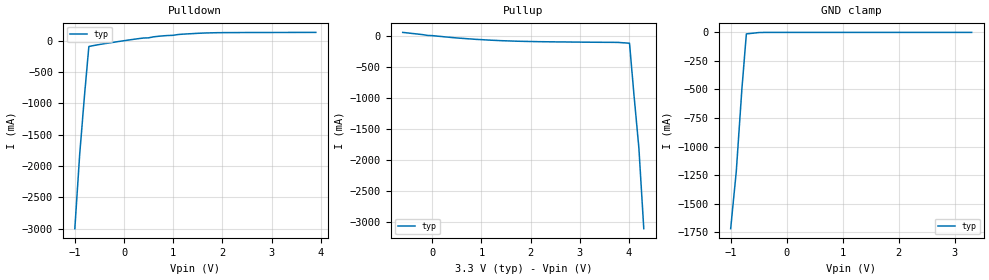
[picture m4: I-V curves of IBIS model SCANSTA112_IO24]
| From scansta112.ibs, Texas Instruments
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|   3-State Output 24mA MODEL
[Model]   SCANSTA112_IO24
Model_type   I/O
Vinh = 2.1
Vinl = 0.8
Vmeas =   1.25
| Variable   typ   min   max
C_comp   5.00pF   NA   NA
|   typ   min   max
[Temperature Range]   25.0   NA   NA
[Voltage range]   3.3V   NA   NA
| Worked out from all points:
|   slope of the pulldown table from 0 to 0.495 V, typ, clamps not added: 10.9 ohm
|   slope of the pullup table from 0 to 0.495 V, typ, clamps not added: 13.5 ohm
|   GND clamp passes 1 mA (typ) near -0.46 V on its own axis
[Pulldown]
| Voltage   I(typ)   I(min)   I(max)
-1V       -3A        NA         NA
-900mV    -1.8A      NA         NA
-800mV    -844mA     NA         NA
-715mV    -93.6mA    NA         NA
300mV     33mA       NA         NA
1.3V      109.2mA    NA         NA
1.9V      127.5mA    NA         NA
3.9V      132.3mA    NA         NA
[Pullup]
| Voltage   I(typ)   I(min)   I(max)
-600mV    52mA       NA         NA
500mV     -37mA      NA         NA
1.4V      -81mA      NA         NA
3.765V    -108.6mA   NA         NA
4.01V     -122mA     NA         NA
4.1V      -947mA     NA         NA
4.2V      -1.8A      NA         NA
4.3V      -3.1A      NA         NA
[GND_clamp]
| Outputs in Tri-state.
| Voltage   I(typ)   I(min)   I(max)
-1V       -1.72A     NA         NA
-900mV    -1.22A     NA         NA
-800mV    -498mA     NA         NA
-720mV    -13mA      NA         NA
-400mV    -240uA     NA         NA
3.3V      586pA      NA         NA
[POWER_clamp]
| Voltage   I(typ)   I(min)   I(max)
-3.3V     0A         NA         NA
3.3V      0A         NA         NA
[Ramp]
|   typ   min   max
dV/dt_r   1.889/1.12n   NA   NA
dV/dt_f   1.889/0.69n   NA   NA
|[Cload]   30p
R_load = 500ohms
